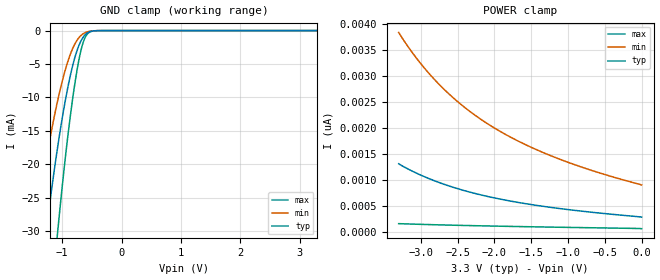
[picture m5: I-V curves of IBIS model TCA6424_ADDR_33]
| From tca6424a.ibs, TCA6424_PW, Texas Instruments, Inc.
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[Model]   TCA6424_ADDR_33
Model_type  Input
Vinl=0.9
Vinh=2.52
| variable   typ   min   max
C_comp   2.21pF   1.76pF   2.42pF
[Temperature Range]   40   100   -40
| Ambient temperature   25   85   -40
[Voltage range]   3.3   3   3.6
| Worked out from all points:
|   GND clamp passes 1 mA (typ) near -0.65 V on its own axis
[GND Clamp]
| TCA6424_ADDR_33
|   Voltage   I(typ)   I(min)   I(max)
-3.3V     -229.8mA   -173.1mA   -314.8mA
-1.49V    -47mA      -31.57mA   -73.96mA
-1.455V   -44.17mA   -29.5mA    -69.9mA
-1.285V   -31.19mA   -20.13mA   -51.01mA
-1.255V   -29.05mA   -18.6mA    -47.84mA
-1.08V    -17.66mA   -10.65mA   -30.52mA
-945mV    -10.37mA   -5.81mA    -18.9mA
-810mV    -4.799mA   -2.428mA   -9.366mA
-700mV    -1.861mA   -882.4uA   -3.61mA
-615mV    -655uA     -320.4uA   -1.07mA
-410mV    -13.36uA   -10.66uA   -11.01uA
3.3V      289.3pA    1.025nA    57.78pA
[POWER Clamp]
| TCA6424_ADDR_33
|   Voltage   I(typ)   I(min)   I(max)
-3.3V     1.315nA    3.842nA    162.7pA
-3.18V    1.219nA    3.582nA    157.1pA
-3.035V   1.119nA    3.303nA    150.7pA
-2.89V    1.03nA     3.055nA    144.8pA
-2.74V    948.5pA    2.827nA    139.1pA
-2.585V   873.6pA    2.616nA    133.6pA
-2.42V    803.1pA    2.417nA    128.2pA
-2.06V    676pA      2.056nA    117.3pA
-1.65V    564.5pA    1.732nA    106.3pA
-1.18V    465.7pA    1.439nA    94.89pA
-640mV    376.5pA    1.169nA    82.73pA
-48.03fV  289.3pA    907.3pA    66.29pA
